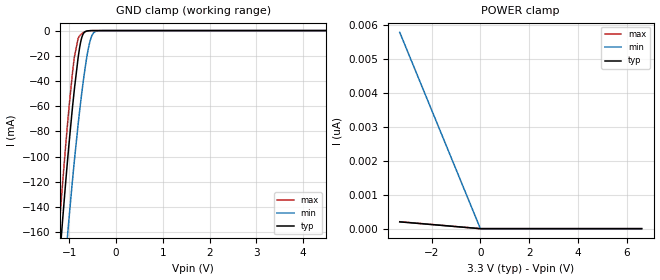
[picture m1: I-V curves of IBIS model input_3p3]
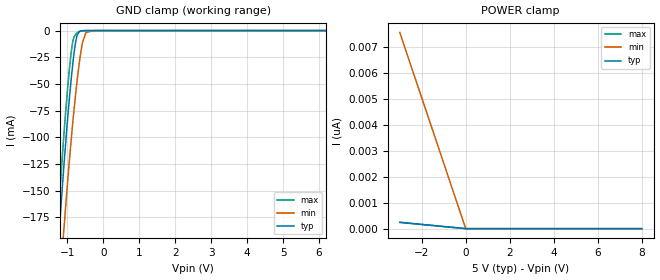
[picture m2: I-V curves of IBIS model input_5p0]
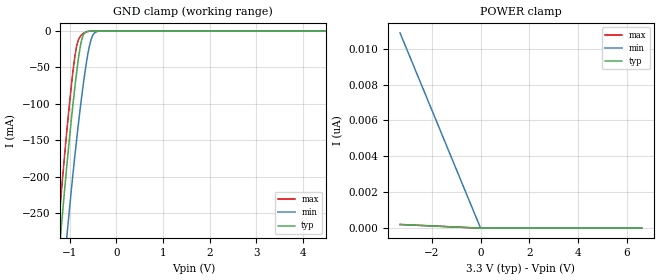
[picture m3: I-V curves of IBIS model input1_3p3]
|Texas Instruments Incorporated
|TLC6C5816-Q1 Power Logic 16-Bit Shift Register LED Driver With Diagnostics
[IBIS Ver]   4.1
[File name]   tlc6c5816-q1.ibs
[Date]   01/07/2019
[File Rev]   1.0
[Source]
| Texas Instruments Incorporated.
| Analog-eLab Design Center, HPA
| 12500 TI Blvd
| Dallas, TX -75243
[Notes]   Revision History:
| Rev 1.0: 01/07/2019
| - Initial version of the model
| - Model generated from simulations in SPECTRE
| - Model names with a trailing _3p3 contain the model for 3.3V operation.
|   Model names with a trailing _5p0 contain the model for 5.0V operation.
| - C_comp although listed in numerical order of value are
|   obtained from varying PVT conditions. For PVT conditions for
|   each specific value refer the buffer description under
|   respective [Model]. IBIS model user is responsible for using
|   appropriate C_comp to simulate for Signal Integrity.
[Disclaimer]
| This model is designed as an aid for customers of Texas Instruments.
| TI and its licensors and suppliers make no warranties, either expressed
| or implied, with respect to this  model, including the warranties of
| merchantability or fitness for a particular purpose. The model is
| provided solely on an "as is" basis. The entire risk as to its quality
| and performance is with the customer.
| This model is subject to change without notice. Texas Instruments
| Incorporated is not responsible for updating this model.
[Copyright]
(C) Copyright 2018 Texas Instruments Incorporated.All rights reserved.
|  Component TLC6C5816-Q1PWP 28-Pin HTSSOP -PWP package
|  Part # TLC6C5816-Q1PWP
[Component]   TLC6C5816-Q1PWP
[Manufacturer]  TI
[Package]   |28 HTSSOP - PWP package
|   typ   min   max
R_pkg   0.05   0.04   0.06
L_pkg   1.0nH   0.8nH   1.2nH
C_pkg   0.2pF   0.16pF   0.24pF
[Pin]  signal_name   model_name   R_pin   L_pin   C_pin
1   VCC   power   NA   NA   NA
2   G1n   input   NA   NA   NA
3   G2n   input   NA   NA   NA
4   DRAIN0   od1   NA   NA   NA
5   DRAIN1/DIAG0   od1   NA   NA   NA
6   DRAIN2   od1   NA   NA   NA
7   DRAIN3/DIAG2   od1   NA   NA   NA
8   DRAIN4   od1   NA   NA   NA
9   DRAIN5/DIAG4   od1   NA   NA   NA
10   DRAIN6   od1   NA   NA   NA
11   DRAIN7/DIAG6   od1   NA   NA   NA
12   SER_IN   input   NA   NA   NA
13   CLRn   input   NA   NA   NA
14   ENn   input1   NA   NA   NA
15   SER_OUT   output   NA   NA   NA
16   RCK   input   NA   NA   NA
17   SRCK   input   NA   NA   NA
18   DRAIN8   od1   NA   NA   NA
19   DRAIN9/DIAG8   od1   NA   NA   NA
20   DRAIN10   od1   NA   NA   NA
21   DRAIN11/DIAG10   od1   NA   NA   NA
22   DRAIN12   od1   NA   NA   NA
23   DRAIN13/DIAG12   od1   NA   NA   NA
24   DRAIN14   od1   NA   NA   NA
25   DRAIN15/DIAG14   od1   NA   NA   NA
26   NC   nc   NA   NA   NA
27   ERRn   od2   NA   NA   NA
28   GND   gnd   NA   NA   NA
|   Model Selectors
[Model Selector] input
input_3p3   3.3V   digital input
input_5p0   5.0V   digital input
[Model Selector] input1
input1_3p3   3.3V   digital input
input1_5p0   5.0V   digital input
[Model Selector] output
output_3p3   3.3V   digital output
output_5p0   5.0V   digital output
[Model Selector] od1
od1_5p5_3p3   5.5V   digital output Open-drain   |VBAT = 5.5V and VCC = 3.3V
od1_12p0_3p3   12.0V   digital output Open-drain   |VBAT = 12.0V and VCC = 3.3V
od1_38p0_3p3   38.0V   digital output Open-drain   |VBAT = 38.0V and VCC = 3.3V
od1_5p5_5p0   5.5V   digital output Open-drain   |VBAT = 5.5V and VCC = 5.0V
od1_12p0_5p0   12.0V   digital output Open-drain   |VBAT = 12.0V and VCC = 5.0V
od1_38p0_5p0   38.0V   digital output Open-drain   |VBAT = 38.0V and VCC = 5.0V
[Model Selector] od2
od2_3p3   3.3V   digital output Open-drain
od2_5p0   5.0V   digital output Open-drain
| Models and submodels in the file (14): input_3p3 (Input), input_5p0 (Input), input1_3p3 (Input), input1_5p0 (Input), output_3p3 (Output), output_5p0 (Output), od1_5p5_3p3 (Open_drain), od1_12p0_3p3 (Open_drain), od1_38p0_3p3 (Open_drain), od1_5p5_5p0 (Open_drain), od1_12p0_5p0 (Open_drain), od1_38p0_5p0 (Open_drain), od2_3p3 (Open_drain), od2_5p0 (Open_drain)
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|   input_3p3 Model
[Model]   input_3p3
Model_type   Input
Vinl = 0.7
Vinh = 2.4
|   typ   min   max
C_comp   1.921pF   1.869pF   1.957pF
|  Where Nom  PVT is Nominal Process, 3.3V,  27C
|   Fast PVT is Strong Process,  3.6V, -40C
|   Slow PVT is Weak Process,   3.0V, 150C
[Voltage Range]   3.3   3   3.6
|Junction Temperature
[Temperature Range]   27   150   -40
[Power Clamp Reference]   3.3   3   3.6
[GND Clamp Reference]   0   0   0
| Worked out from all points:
|   GND clamp passes 1 mA (typ) near -0.67 V on its own axis
[GND Clamp]
|   Voltage   I(typ)   I(min)   I(max)
-3.3V     -1.285A    -1.281A    -1.297A
-1.27V    -209.6mA   -266.1mA   -181.8mA
-1.191V   -171.1mA   -229.3mA   -142.2mA
-1.152V   -152.3mA   -211.3mA   -123.1mA
-1.043V   -103.4mA   -163mA     -74.42mA
-894.3mV  -46.16mA   -102.8mA   -20.7mA
-815.1mV  -21.56mA   -74.43mA   -6.284mA
-775.5mV  -12mA      -61.42mA   -3.857mA
-666.6mV  -961.9uA   -29.99mA   -870.1uA
-537.9mV  -39.91uA   -5.667mA   -45.17uA
-399.3mV  -772.3nA   -213.4uA   -436.5nA
6.6V      0A         0A         0A
[POWER Clamp]
|   Voltage   I(typ)   I(min)   I(max)
-3.3V     200.5pA    5.789nA    205.2pA
0V        0A         0A         0A
6.6V      0A         0A         0A
|   input_5p0 Model
[Model]   input_5p0
Model_type   Input
Vinl = 0.7
Vinh = 2.4
|   typ   min   max
C_comp   1.769pF   1.72pF   1.785pF
|  Where Nom  PVT is Nominal Process, 5.0V,  27C
|   Fast PVT is Strong Process,  5.5V, -40C
|   Slow PVT is Weak Process,   4.5V, 150C
[Voltage Range]   5   4.5   5.5
|Junction Temperature
[Temperature Range]   27   150   -40
[Power Clamp Reference]   5   4.5   5.5
[GND Clamp Reference]   0   0   0
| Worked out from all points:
|   GND clamp passes 1 mA (typ) near -0.67 V on its own axis
[GND Clamp]
|   Voltage   I(typ)   I(min)   I(max)
-3V       -1.123A    -1.128A    -1.129A
-1.537V   -344.9mA   -393.7mA   -322.2mA
-1.229V   -189.2mA   -246.7mA   -160.8mA
-1.097V   -127.2mA   -186.7mA   -97.87mA
-899mV    -47.78mA   -104.5mA   -22.02mA
-844mV    -29.87mA   -84.42mA   -9.678mA
-767mV    -10.3mA    -58.73mA   -3.499mA
-668mV    -996.6uA   -30.34mA   -891.8uA
-580mV    -114.2uA   -11.42mA   -135.4uA
-481mV    -8.852uA   -1.671mA   -8.456uA
-239mV    0A         -3.044uA   0A
8V        0A         0A         0A
[POWER Clamp]
|   Voltage   I(typ)   I(min)   I(max)
-3V       240.9pA    7.575nA    247.6pA
0V        0A         0A         0A
8V        0A         0A         0A
|   input1_3p3 Model
[Model]   input1_3p3
Model_type   Input
Vinl = 0.7
Vinh = 2.4
|   typ   min   max
C_comp   3.799pF   3.712pF   3.869pF
|  Where Nom  PVT is Nominal Process, 3.3V,  27C
|   Fast PVT is Strong Process,  3.6V, -40C
|   Slow PVT is Weak Process,   3.0V, 150C
[Voltage Range]   3.3   3   3.6
|Junction Temperature
[Temperature Range]   27   150   -40
[Power Clamp Reference]   3.3   3   3.6
[GND Clamp Reference]   0   0   0
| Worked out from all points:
|   GND clamp passes 1 mA (typ) near -0.64 V on its own axis
[GND Clamp]
|   Voltage   I(typ)   I(min)   I(max)
-3.3V     -2.023A    -2.04A     -2.027A
-1.28V    -344.5mA   -438.9mA   -298.3mA
-1.221V   -299mA     -395.1mA   -251.9mA
-1.162V   -254.8mA   -352.1mA   -207.1mA
-1.063V   -184.5mA   -282.4mA   -136.8mA
-894.3mV  -78.93mA   -173.3mA   -36.45mA
-854.7mV  -57.43mA   -149.9mA   -21.05mA
-765.6mV  -18.35mA   -100.8mA   -6.724mA
-646.8mV  -1.151mA   -44.86mA   -1.183mA
-518.1mV  -46.34uA   -7.333mA   -50.25uA
-359.7mV  -368nA     -146.7uA   -115.5nA
6.6V      0A         0A         0A
[POWER Clamp]
|   Voltage   I(typ)   I(min)   I(max)
-3.3V     203.2pA    10.88nA    205.2pA
0V        0A         0A         0A
6.6V      0A         0A         0A
